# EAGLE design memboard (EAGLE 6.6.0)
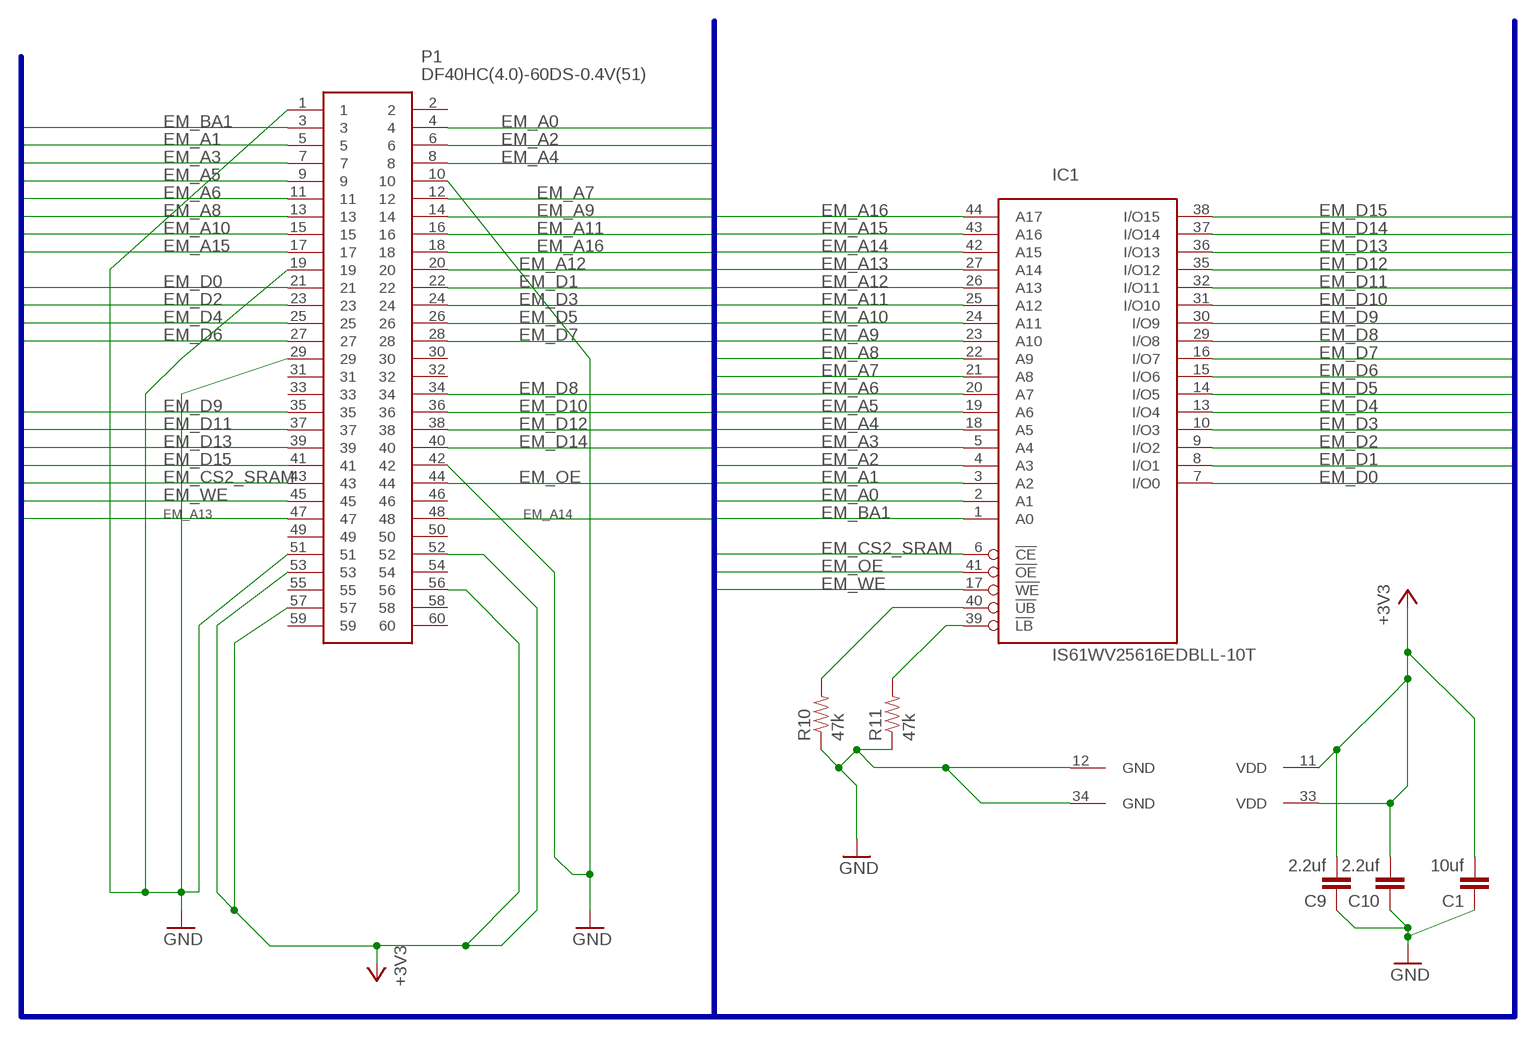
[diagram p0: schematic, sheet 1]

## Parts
C1  10uf  CAP0805  [0805]
C9  2.2uf  CAP0805  [0805]
C10  2.2uf  CAP0805  [0805]
IC1  IS61WV25616EDBLL-10T  [TSOP-II-44]
P1  DF40HC(4.0)-60DS-0.4V(51)  [DF40HC4060DS04V51]
R10  47k  RESISTOR0805-RES  [0805]
R11  47k  RESISTOR0805-RES  [0805]

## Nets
+3V3 [power]: C1.2 C9.2 C10.2 IC1.11(VDD) IC1.33(VDD) P1.52 P1.53 P1.56 P1.57
EM_A0: IC1.2(A1) P1.4
EM_A1: IC1.3(A2) P1.5
EM_A2: IC1.4(A3) P1.6
EM_A3: IC1.5(A4) P1.7
EM_A4: IC1.18(A5) P1.8
EM_A5: IC1.19(A6) P1.9
EM_A6: IC1.20(A7) P1.11
EM_A7: IC1.21(A8) P1.12
EM_A8: IC1.22(A9) P1.13
EM_A9: IC1.23(A10) P1.14
EM_A10: IC1.24(A11) P1.15
EM_A11: IC1.25(A12) P1.16
EM_A12: IC1.26(A13) P1.20
EM_A13: IC1.27(A14) P1.47
EM_A14: IC1.42(A15) P1.48
EM_A15: IC1.43(A16) P1.17
EM_A16: IC1.44(A17) P1.18
EM_BA1: IC1.1(A0) P1.3
EM_CS2_SRAM: IC1.6(!CE) P1.43
EM_D0: IC1.7(I/O0) P1.21
EM_D1: IC1.8(I/O1) P1.22
EM_D2: IC1.9(I/O2) P1.23
EM_D3: IC1.10(I/O3) P1.24
EM_D4: IC1.13(I/O4) P1.25
EM_D5: IC1.14(I/O5) P1.26
EM_D6: IC1.15(I/O6) P1.27
EM_D7: IC1.16(I/O7) P1.28
EM_D8: IC1.29(I/O8) P1.34
EM_D9: IC1.30(I/O9) P1.35
EM_D10: IC1.31(I/O10) P1.36
EM_D11: IC1.32(I/O11) P1.37
EM_D12: IC1.35(I/O12) P1.38
EM_D13: IC1.36(I/O13) P1.39
EM_D14: IC1.37(I/O14) P1.40
EM_D15: IC1.38(I/O15) P1.41
EM_OE: IC1.41(!OE) P1.44
EM_WE: IC1.17(!WE) P1.45
GND [power]: C1.1 C9.1 C10.1 IC1.12(GND) IC1.34(GND) P1.1 P1.10 P1.19 P1.29 P1.42 P1.51 R10.1 R11.1
N$1: IC1.40(!UB) R10.2
N$2: IC1.39(!LB) R11.2
Unconnected: P1.2 P1.30 P1.31 P1.32 P1.33 P1.46 P1.49 P1.50 P1.54 P1.55 P1.58 P1.59 P1.60

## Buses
BUS:EM_BA1,EM_A[0..16],EM_D[0..15],EM_CS2_SRAM,EM_OE,EM_WE

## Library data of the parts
C1 C9 C10 = SparkFun-Capacitors:CAP: Capacitor
IC1 = memory-issi-asynsram:IS61WV25616EDBLL-*: 256k x 16 high- speed CMOS static RAM with ECC 8ns and 10ns access time 3.6V power supply
P1 = DF40HC(4.0)-60DS-0.4V(51):DF40HC(4.0)-60DS-0.4V(51): HIROSE(HRS) - DF40HC(4.0)-60DS-0.4V(51) - CONNECTOR, STACKING, RCPT, 60POS, 2ROW Source: Datasheet; DESCRIPTION: HIROSE(HRS) - DF40HC(4.0)-60DS-0.4V(51) - CONNECTOR, STACKING, RCPT, 60POS, 2ROW; HEIGHT: 4.05mm; MANUFACTURER_NAME: Hirose; MANUFACTURER_PART_NUMBER: DF40HC(4.0)-60DS-0.4V(51); MOUSER_PART_NUMBER: 798-DF4HC4060DS04V51; MOUSER_PRICE-STOCK: https://www.mouser.com/Search/Refine.aspx?Keyword=798-DF4HC4060DS04V51
R10 R11 = SparkFun-Resistors:RESISTOR: Resistor

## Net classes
0 default: width 0.178 mm, drill 0.127 mm, clearance 0.178 mm
1 power: width 0.254 mm, drill 0.127 mm, clearance 0.152 mm

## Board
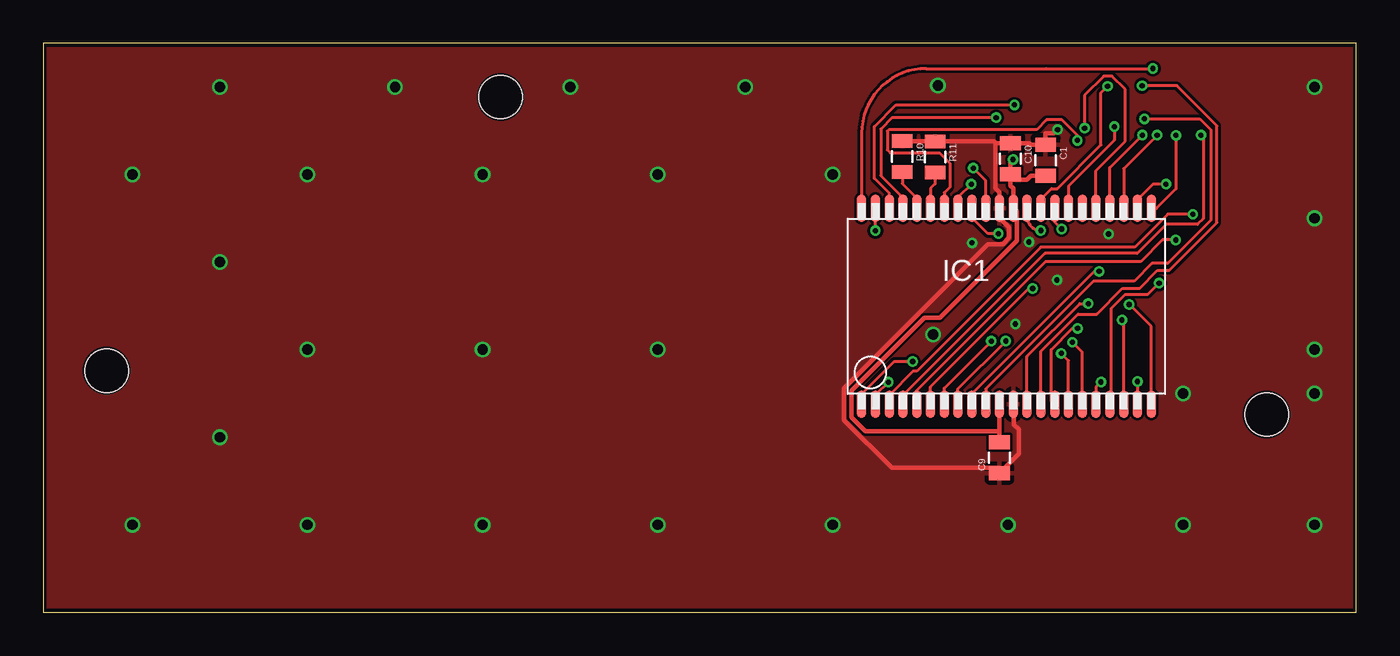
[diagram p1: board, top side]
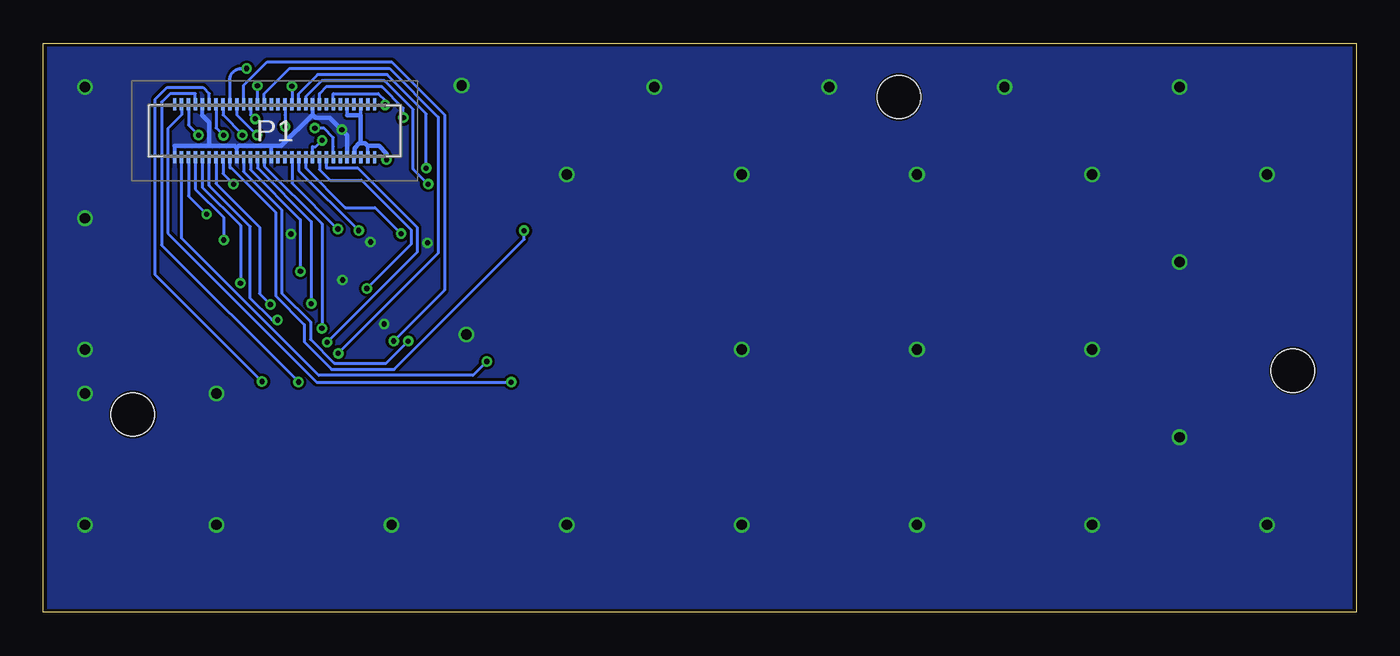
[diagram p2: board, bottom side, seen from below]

Size 76.2 x 33.02 mm. Coordinates in mm from the lower left corner, seen from the top.
Outline: 0,0 76.2,0 76.2,33.02 0,33.02 0,0
Copper layers (1*16): Top 0.035mm / dielectric 1.5mm / Bottom 0.035mm
Design rules "memboard": minimum track width 5mil, minimum drill 0.3mm, track to track 5mil, track to pad 5mil, pad to pad 5mil, via to via 5mil, smd to smd 5mil, copper to edge 5mil, drill to drill 5mil, minimum pad ring 6mil, minimum via ring 6mil, stop-mask expansion 4mil, vias tented up to drill 25mil, thermal gap 10mil
Holes 2.5 mm at 70.99,11.48 26.54,29.9 3.68,14.02

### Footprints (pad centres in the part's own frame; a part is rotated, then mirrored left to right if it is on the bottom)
0805 = smd 0.8 x 1.2: 1 -0.9,0; 2 0.9,0
TSOP-II-44 = smd 0.55 x 1.6: 1 -8.4,-5.68; 2 -7.6,-5.68; 3 -6.8,-5.68; 4 -6,-5.68; 5 -5.2,-5.68; 6 -4.4,-5.68; 7 -3.6,-5.68; 8 -2.8,-5.68; 9 -2,-5.68; 10 -1.2,-5.68; 11 -0.4,-5.68; 12 0.4,-5.68; 13 1.2,-5.68; 14 2,-5.68; 15 2.8,-5.68; 16 3.6,-5.68; 17 4.4,-5.68; 18 5.2,-5.68; 19 6,-5.68; 20 6.8,-5.68; 21 7.6,-5.68; 22 8.4,-5.68; 23 8.4,5.68; 24 7.6,5.68; 25 6.8,5.68; 26 6,5.68; 27 5.2,5.68; 28 4.4,5.68; 29 3.6,5.68; 30 2.8,5.68; 31 2,5.68; 32 1.2,5.68; 33 0.4,5.68; 34 -0.4,5.68; 35 -1.2,5.68; 36 -2,5.68; 37 -2.8,5.68; 38 -3.6,5.68; 39 -4.4,5.68; 40 -5.2,5.68; 41 -6,5.68; 42 -6.8,5.68; 43 -7.6,5.68; 44 -8.4,5.68
DF40HC4060DS04V51 = smd 0.2 x 0.7: 1 -5.8,-1.54; 2 -5.8,1.54; 3 -5.4,-1.54; 4 -5.4,1.54; 5 -5,-1.54; 6 -5,1.54; 7 -4.6,-1.54; 8 -4.6,1.54; 9 -4.2,-1.54; 10 -4.2,1.54; 11 -3.8,-1.54; 12 -3.8,1.54; 13 -3.4,-1.54; 14 -3.4,1.54; 15 -3,-1.54; 16 -3,1.54; 17 -2.6,-1.54; 18 -2.6,1.54; 19 -2.2,-1.54; 20 -2.2,1.54; 21 -1.8,-1.54; 22 -1.8,1.54; 23 -1.4,-1.54; 24 -1.4,1.54; 25 -1,-1.54; 26 -1,1.54; 27 -0.6,-1.54; 28 -0.6,1.54; 29 -0.2,-1.54; 30 -0.2,1.54; 31 0.2,-1.54; 32 0.2,1.54; 33 0.6,-1.54; 34 0.6,1.54; 35 1,-1.54; 36 1,1.54; 37 1.4,-1.54; 38 1.4,1.54; 39 1.8,-1.54; 40 1.8,1.54; 41 2.2,-1.54; 42 2.2,1.54; 43 2.6,-1.54; 44 2.6,1.54; 45 3,-1.54; 46 3,1.54; 47 3.4,-1.54; 48 3.4,1.54; 49 3.8,-1.54; 50 3.8,1.54; 51 4.2,-1.54; 52 4.2,1.54; 53 4.6,-1.54; 54 4.6,1.54; 55 5,-1.54; 56 5,1.54; 57 5.4,-1.54; 58 5.4,1.54; 59 5.8,-1.54; 60 5.8,1.54

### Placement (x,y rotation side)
C1  0.1uf  [0805]  58.17,26.23 270 top
C9  55.49,8.97 90 top
C10  56.12,26.31 270 top
IC1  55.89,17.75 0 top
P1  62.76,27.94 0 bottom
R10  49.85,26.44 270 top
R11  51.75,26.42 270 top

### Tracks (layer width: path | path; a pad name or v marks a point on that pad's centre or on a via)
+3V3  (via drill 0.3 pad 0.6)
  Top 0.254: 55.49,10.52 47.7,10.52 46.91,11.31 46.91,12.86 51.14,17.09 52.03,17.09 56.49,21.55 56.49,23.19 56.49,23.24 arc90 IC1.33 56.29,24.59 56.12,24.76 56.12,25.09 | v56.28,26.27 56.28,26.22 56.12,26.07 C10.2 56.12,25.09 | C9.2 55.49,10.52 | 55.49,10.52 IC1.11 | C1.2 57.31,25.33 57.07,25.09 56.12,25.09
  Bottom 0.025: P1.53 58.14,26.4
  Bottom 0.2: 58.56,28.83 P1.52 | 57.76,28.83 P1.56 | 57.36,27.05 P1.57
  Bottom 0.254: v56.28,26.27 56.28,26.61 56.72,27.05 57.36,27.05 57.51,27.2 57.76,27.2 | 58.56,28.83 57.76,28.83 57.76,27.2 | 57.76,27.2 57.86,27.2 58.14,26.92 58.14,26.4
EM_A0  (via drill 0.3 pad 0.6)
  Top 0.178: v49.04,13.36 48.29,12.61 IC1.2
  Bottom 0.178: v49.04,13.36 60.33,13.36 68.97,21.99 68.97,28.06 68.16,28.86 P1.4
EM_A1  (via drill 0.3 pad 0.6)
  Top 0.178: v66.71,23.09 65.25,23.09 63.34,21.18 57.89,21.18 50.69,13.99 50.48,13.99 49.09,12.6 IC1.3
  Bottom 0.178: P1.5 67.76,24.15 v66.71,23.09
EM_A2  (via drill 0.3 pad 0.6)
  Top 0.178: v67.18,27.68 67.31,27.54 67.31,22.84 66.97,22.5 65.16,22.5 63.49,20.83 58.14,20.83 49.89,12.58 IC1.4
  Bottom 0.178: P1.6 67.76,28.27 v67.18,27.68
EM_A3  (via drill 0.3 pad 0.6)
  Top 0.178: v65.72,21.6 64.94,21.6 63.69,20.35 58.16,20.35 50.69,12.88 IC1.5
  Bottom 0.178: P1.7 67.36,24.55 65.72,22.91 v65.72,21.6
EM_A4  (via drill 0.3 pad 0.6)
  Top 0.178: v61.38,13.37 61.09,13.08 IC1.18 | IC1.18
  Bottom 0.178: P1.8 67.36,30.1 68.82,30.1 69.32,29.6 69.32,21.31 v61.38,13.37
EM_A5  (via drill 0.3 pad 0.6)
  Top 0.178: IC1.19 61.99,12.17 61.99,17.64 62.79,18.44 64.1,18.44 v64.75,19.09
  Bottom 0.178: P1.9 66.96,24.66 64.75,22.44 v64.75,19.09
EM_A6  (via drill 0.3 pad 0.6)
  Top 0.178: IC1.20 62.69,16.86 v62.6,16.96
  Bottom 0.178: v62.6,16.96 62.92,16.96 64.18,18.22 64.18,22.38 66.56,24.76 P1.11
EM_A7  (via drill 0.3 pad 0.6)
  Top 0.178: v63.49,13.39 IC1.21
  Bottom 0.178: v63.49,13.39 69.7,19.6 69.7,29.75 69,30.45 66.92,30.45 66.56,30.1 P1.12
EM_A8  (via drill 0.3 pad 0.6)
  Top 0.178: IC1.22 | IC1.22 64.29,16.58 v63.01,17.86
  Bottom 0.178: P1.13 66.16,24.86 63.64,22.34 63.64,18.49 v63.01,17.86
EM_A9  (via drill 0.3 pad 0.6)
  Top 0.178: v65.73,27.67 65.73,24.56 64.6,23.44 IC1.23
  Bottom 0.178: P1.14 66.16,28.1 v65.73,27.67
EM_A10  (via drill 0.3 pad 0.6)
  Top 0.178: v65.15,24.84 64.39,24.84 63.49,23.94 IC1.24
  Bottom 0.178: P1.15 65.76,25.46 v65.15,24.84
EM_A11  (via drill 0.3 pad 0.6)
  Top 0.178: v64.64,27.68 62.69,25.74 IC1.25
  Bottom 0.178: v64.64,27.68 64.64,27.74 65.76,28.86 P1.16
EM_A12  (via drill 0.3 pad 0.6)
  Top 0.178: IC1.26 61.89,25.79 v63.78,27.68
  Bottom 0.178: v63.78,27.68 64.96,28.86 P1.20
EM_A13  (via drill 0.3 pad 0.6)
  Top 0.178: IC1.27 61.09,25.63 62.79,27.33 62.79,30.33 62.02,31.1 61.54,31.1 60.43,29.99 v60.43,28.08
  Bottom 0.178: v60.43,28.08 59.9,28.08 59.36,27.54 59.36,27.02 P1.47
EM_A14  (via drill 0.3 pad 0.6)
  Top 0.178: IC1.42 49.09,24.31 48.23,25.17 48.23,28.18 49.49,29.44 v56.35,29.44
  Bottom 0.178: v56.35,29.44 56.35,29.7 56.75,30.1 59.36,30.1 P1.48
EM_A15  (via drill 0.3 pad 0.6)
  Top 0.178: v48.29,22.14 IC1.43
  Bottom 0.178: v48.29,22.14 48.29,21.64 55.83,14.1 59.46,14.1 61.04,15.69 61.04,16.7 62.71,18.36 62.71,23.2 65.29,25.78 65.36,25.78 P1.17
EM_A16  (via drill 0.3 pad 0.6)
  Top 0.178: v64.39,31.55 58.19,31.55 51.23,31.55 arc90 47.49,27.81 IC1.44
  Bottom 0.178: P1.18 65.36,30.88 arc90 64.69,31.55 v64.39,31.55
EM_BA1  (via drill 0.3 pad 0.6)
  Top 0.178: IC1.1 47.49,12.66 49.39,14.56 v50.45,14.56
  Bottom 0.178: v50.45,14.56 51.26,13.75 60.21,13.75 68.16,21.7 P1.3
EM_CS2_SRAM  (via drill 0.3 pad 0.6)
  Top 0.178: IC1.6 51.49,13.09 57.19,18.79 v57.41,18.79
  Bottom 0.178: P1.43 60.16,25.68 59.55,25.07 57.73,25.07 54.86,22.2 54.86,21.34 v57.41,18.79
EM_D0  (via drill 0.3 pad 0.6)
  Top 0.178: IC1.7 52.29,13.01 v55.02,15.74
  Bottom 0.178: P1.21 64.56,25.56 62.35,23.35 62.35,18.51 60.69,16.84 60.69,15.83 59.31,14.46 56.3,14.46 v55.02,15.74
EM_D1  (via drill 0.3 pad 0.6)
  Top 0.178: IC1.8 53.09,12.97 v55.86,15.74
  Bottom 0.178: P1.22 64.56,30.56 63.19,31.93 55.98,31.93 52.91,28.87 52.91,18.69 v55.86,15.74
EM_D2  (via drill 0.3 pad 0.6)
  Top 0.178: v61.28,19.78 60.99,19.78 53.89,12.68 IC1.9
  Bottom 0.178: P1.23 64.16,25.68 61.28,22.79 v61.28,19.78
EM_D3  (via drill 0.3 pad 0.6)
  Top 0.178: v63.9,28.63 67.11,28.63 67.76,27.98 67.76,22.76 65.24,20.24 64.34,20.24 63.31,19.21 60.94,19.21 54.69,12.96 IC1.10
  Bottom 0.178: P1.24 64.16,28.86 64.13,28.86 v63.9,28.63
EM_D4  (via drill 0.3 pad 0.6)
  Top 0.178: IC1.13 57.09,14.85 60.15,17.91 v60.64,17.91
  Bottom 0.178: v60.64,17.91 60.64,22.66 63.76,25.78 P1.25
EM_D5  (via drill 0.3 pad 0.6)
  Top 0.178: IC1.14 57.89,15.15 60.05,17.31 61.13,17.31 62.62,18.8 63.62,18.8 64.66,19.84 65.34,19.84 68.11,22.61 68.11,28.22 65.78,30.55 v63.76,30.55
  Bottom 0.178: P1.26 v63.76,30.55
EM_D6  (via drill 0.3 pad 0.6)
  Top 0.178: IC1.15 58.49,12.27 58.49,15.25 59.72,16.47 v60.02,16.47
  Bottom 0.178: P1.27 63.36,25.88 60.02,22.54 v60.02,16.47
EM_D7  (via drill 0.3 pad 0.6)
  Top 0.178: IC1.16 59.49,14.61 v59.08,15.03
  Bottom 0.178: v59.08,15.03 53.27,20.83 53.27,28.72 56.1,31.56 61.9,31.56 63.36,30.1 P1.28
EM_D8  (via drill 0.3 pad 0.6)
  Top 0.178: v62.15,28.17 62.15,27.39 59.49,24.72 IC1.29
  Bottom 0.178: v62.15,28.17 62.15,28.85 62.16,28.86 P1.34
EM_D9  (via drill 0.3 pad 0.6)
  Top 0.178: v59.1,22.23 58.69,22.64 IC1.30
  Bottom 0.178: P1.35 61.76,24.9 v59.1,22.23
EM_D10  (via drill 0.3 pad 0.6)
  Top 0.178: IC1.31 57.89,23.97 58.51,24.58 58.85,24.58 61.39,27.12 61.39,30.14 v61.76,30.52
  Bottom 0.178: v61.76,30.52 P1.36
EM_D11  (via drill 0.3 pad 0.6)
  Top 0.178: IC1.32 57.09,22.95 arc90 v57.89,22.15
  Bottom 0.178: P1.37 61.36,25.63 v57.89,22.15
EM_D12  (via drill 0.3 pad 0.6)
  Top 0.178: IC1.35 54.69,25.04 v53.97,25.77
  Bottom 0.178: v53.97,25.77 53.97,28.92 56.24,31.19 60.27,31.19 61.36,30.1 P1.38
EM_D13  (via drill 0.3 pad 0.6)
  Top 0.178: v55.43,21.97 54.82,21.97 53.89,22.89 IC1.36
  Bottom 0.178: P1.39 60.96,25.78 58.66,23.48 56.94,23.48 v55.43,21.97
EM_D14  (via drill 0.3 pad 0.6)
  Top 0.178: v53.86,24.84 53.09,24.07 IC1.37
  Bottom 0.178: v53.86,24.84 54.73,25.71 54.73,29.18 56.39,30.83 60.05,30.83 60.96,29.92 P1.40
EM_D15  (via drill 0.3 pad 0.6)
  Top 0.178: v60.01,27.38 60.01,27.69 59.12,28.57 58.22,28.57 57.66,28.01 49.08,28.01 48.98,27.91 48.98,26.83 49.16,26.65 52.01,26.65 52.62,26.04 52.62,24.67 52.29,24.34 IC1.38
  Bottom 0.178: P1.41 60.56,27.02 60.37,27.02 v60.01,27.38
EM_OE  (via drill 0.3 pad 0.6)
  Top 0.178: v55.3,28.69 49.26,28.69 48.6,28.03 48.6,25.34 49.89,24.05 IC1.41
  Bottom 0.178: v55.3,28.69 55.3,29.24 56.53,30.47 59.79,30.47 60.16,30.1 P1.44
EM_WE  (via drill 0.3 pad 0.6)
  Top 0.178: IC1.17 60.29,15.1 v59.72,15.67
  Bottom 0.178: v59.72,15.67 54.5,20.89 54.5,22.35 57.94,25.78 59.76,25.78 P1.45
GND  (via drill 0.3, 0.3 pad 0.6, 0.6)
  Top 0.254: 55.24,27.21 55.24,24.61 55.49,24.36 IC1.34 55.49,22.9 56.05,22.34 56.05,21.72 55.68,21.36 54.82,21.36 46.47,13.02 46.47,11.16 49.24,8.39 55.49,8.39 C9.1 56.62,9.2 56.62,10.62 56.34,10.89 56.34,12.03 IC1.12 | 55.24,27.21 55.36,27.21 C10.1 57.22,27.21 57.31,27.13 C1.1 58.17,27.78 58.65,27.78 v58.87,28 | R10.1 50.7,27.34 50.73,27.32 R11.1 55.14,27.32 arc-90 55.24,27.21
  Bottom 0.2: 66.96,28.83 P1.10 | P1.51 | 60.56,28.87 P1.42 | 68.56,27.05 P1.1 | 64.96,26.93 P1.19 | 62.96,27.05 P1.29
  Bottom 0.254: 66.56,27.05 68.56,27.05 | 66.56,27.05 65.09,27.05 64.96,26.93 64.84,27.05 62.96,27.05 62.38,27.05 60.56,28.87 60.39,28.7 59.57,28.7 v58.87,28 58.57,27.69 P1.51 | 66.56,27.05 66.56,28.42 66.96,28.83
  other vias: 51.92,30.56 58.83,19.28 51.64,16.13 5.18,5.08 15.34,5.08 25.5,5.08 35.66,5.08 45.82,5.08 55.98,5.08 66.14,5.08 66.14,12.7 73.76,12.7 15.34,15.24 15.34,25.4 5.18,25.4 25.5,25.4 25.5,15.24 35.66,15.24 35.66,25.4 45.82,25.4 40.74,30.48 30.58,30.48 20.42,30.48 10.26,30.48 10.26,20.32 10.26,10.16 73.76,22.86 73.76,30.48 73.76,5.08 73.76,15.24 57.2,21.49 56.41,16.73 61.82,21.95 53.9,21.44
  pour Bottom (isolate 0.127): 0.23,32.79 75.97,32.79 75.97,0.23 0.23,0.23
  pour Top (isolate 0.127): 0.23,32.79 75.97,32.79 75.97,0.23 0.23,0.23
N$1
  Top 0.178: R10.2 49.85,24.88 50.69,24.03 IC1.40
N$2
  Top 0.178: R11.2 51.75,24.85 51.49,24.59 IC1.39

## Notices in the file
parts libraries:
SparkFun-Resistors: Licensing: Creative Commons ShareAlike 4.0 International - https://creativecommons.org/licenses/by-sa/4.0
